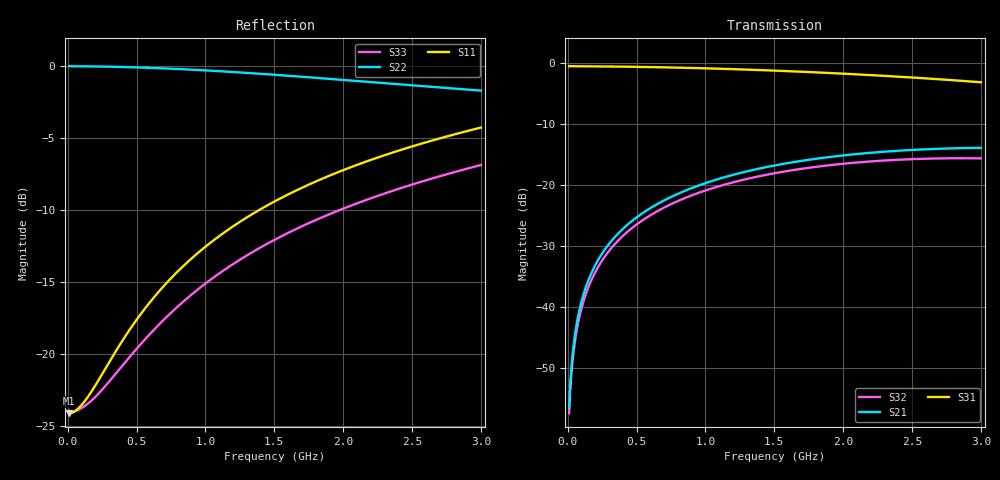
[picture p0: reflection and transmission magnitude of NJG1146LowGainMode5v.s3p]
! Created Mon Oct 18 18:41:05 2010
# hz S ma R 50
! 3 Port Network Data Port1:RFIN  Port2:RFOUT1  Port3:RFOUT2
! freq  magS11  angS11  magS12  angS12  magS13  angS13
!  magS21  angS21
!  magS22  angS22  magS23  angS23
!  magS31  angS31  magS32  angS32
!  magS33  angS33
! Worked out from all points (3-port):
!   2991 points, 10 MHz to 3 GHz, reference 50 ohm
!   strongest paths, dB at 10 MHz, 757 MHz, 1.505 GHz, 2.253 GHz, 3 GHz:
!     S31: -0.6, -0.8, -1.3, -2.1, -3.2
!     S21: -56.5, -22.0, -16.9, -14.7, -14.0
!     S32: -57.5, -23.1, -18.1, -16.1, -15.7
!   lowest |S11| = -24.1 dB at 10 MHz (marker M1), VSWR 1.13, Z = 56.6 - j0.31 ohm
!   |S11| at or under -10 dB: start of sweep to 1.393 GHz
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1e7  0.0621 -2.5  0.001486 69.4  0.9346 -0.2
     0.001495 69.8  0.9968 -0.4  0.00134 69.6
     0.9346 -0.2  0.001332 69.2  0.06249 -2.0
5.1e7  0.06312 -12.5  0.005632 80.5  0.9341 -1.2
       0.00572 80.7  0.9959 -1.4  0.005111 80.7
       0.9341 -1.2  0.005034 80.5  0.06308 -9.6
1.08e8  0.06698 -25.3  0.01167 82.5  0.9332 -2.4
        0.01187 82.6  0.9956 -3.0  0.01059 82.6
        0.9332 -2.4  0.01042 82.5  0.06509 -19.8
2.01e8  0.07768 -42.6  0.02159 80.9  0.9314 -4.5
        0.02195 81.0  0.9944 -5.6  0.01957 81.1
        0.9314 -4.5  0.01925 81.0  0.07085 -34.7
3.37e8  0.09986 -60.2  0.03598 76.9  0.9281 -7.4
        0.03658 76.9  0.9918 -9.3  0.03258 77.2
        0.9281 -7.4  0.03205 77.2  0.08398 -52.0
5.33e8  0.1379 -76.3  0.05627 70.5  0.9215 -11.7
        0.05722 70.5  0.9861 -14.6  0.05088 70.9
        0.9215 -11.7  0.05004 70.9  0.1084 -69.7
7.9e8  0.1913 -89.9  0.08165 61.8  0.9098 -17.2
       0.08303 61.8  0.9751 -21.5  0.07367 62.5
       0.9098 -17.2  0.07245 62.5  0.1446 -85.6
1.505e9  0.3386 -114.3  0.1412 37.9  0.8591 -32.2
         0.1436 37.9  0.9303 -40.1  0.1262 39.2
         0.8592 -32.2  0.124 39.2  0.2491 -114.2
2.219e9  0.4744 -132.6  0.1799 15.0  0.7875 -46.9
         0.183 15.0  0.8762 -57.5  0.158 16.9
         0.7875 -46.9  0.1553 16.9  0.349 -135.3
3e9  0.6101 -150.3  0.1964 -9.1  0.6897 -62.9
     0.2 -9.1  0.8199 -75.6  0.167 -6.3
     0.6897 -62.9  0.164 -6.3  0.4522 -155.7
